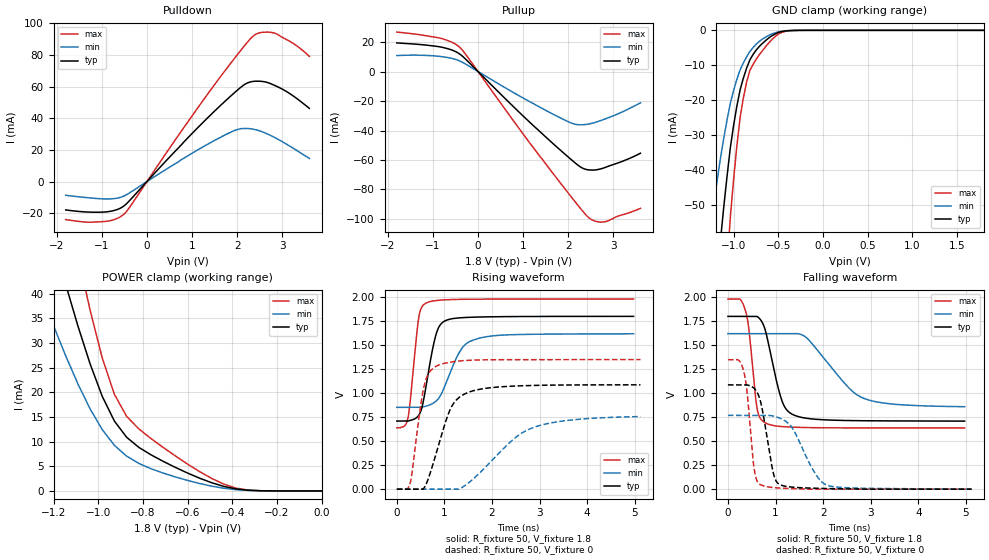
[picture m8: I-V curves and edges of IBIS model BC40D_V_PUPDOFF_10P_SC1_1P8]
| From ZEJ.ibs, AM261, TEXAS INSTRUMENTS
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[Model]   BC40D_V_PUPDOFF_10P_SC1_1P8
Model_type   I/O
Polarity   Non-Inverting
Enable   Active-Low
Vinl =  0.63
Vinh =  1.17
Cref =  15pF
Rref =  100.0000M
Vref =  0V
Vmeas =  0.9
C_comp   2.290246p   2.205796p   2.292736p
|[Input load] weak_pupdoff
|[Output drive] slow
|[supplytol] 10
|[temp] ind
[Model Spec]
Vinl   0.63   0.567   0.693
Vinh   1.17   1.053   1.287
[Temperature Range]   25   125   -40
[Voltage Range]   1.8   1.62   1.98
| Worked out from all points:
|   slope of the pulldown table from 0 to 0.27 V, typ, clamps not added: 32.2 ohm
|   slope of the pullup table from 0 to 0.27 V, typ, clamps not added: 32.6 ohm
|   GND clamp passes 1 mA (typ) near -0.53 V on its own axis
|   POWER clamp passes 1 mA (typ) near -0.44 V on its own axis
|   rising waveform, R_fixture 50, V_fixture 1.8: 20-80 % time 246ps typ, 417ps min, 160ps max; typ from 0.709 V to 1.8 V
|   rising waveform, R_fixture 50, V_fixture 0: 20-80 % time 429ps typ, 995ps min, 230ps max; typ from 0 V to 1.09 V
|   falling waveform, R_fixture 50, V_fixture 1.8: 20-80 % time 308ps typ, 788ps min, 165ps max; typ from 1.8 V to 0.709 V
|   falling waveform, R_fixture 50, V_fixture 0: 20-80 % time 226ps typ, 462ps min, 150ps max; typ from 1.09 V to 0 V
| Nom Voltages:
|   VDD=1.1001, VDDS=1.8, VDDS18=1.8, ESD_BIASFET=0, VSS=0, VSSS=0
| Min Voltages:
|   VDD=0.99, VDDS=1.62, VDDS18=1.62, ESD_BIASFET=0, VSS=0, VSSS=0
| Max Voltages:
|   VDD=1.21, VDDS=1.98, VDDS18=1.98, ESD_BIASFET=0, VSS=0, VSSS=0
[POWER_clamp]
|   voltage   I(typ)   I(min)   I(max)
-1.8V     158.8mA    112.5mA    219.7mA
-1.255V   59.93mA    40mA       84.85mA
-1.127V   39.08mA    25.51mA    55.74mA
-1.055V   28.36mA    18.34mA    40.4mA
-981.8mV  19.18mA    12.43mA    26.97mA
-927.3mV  14.16mA    9.242mA    19.58mA
-872.7mV  10.89mA    7.052mA    15.14mA
-818.2mV  8.843mA    5.581mA    12.58mA
-600mV    3.63mA     2.129mA    5.448mA
-436.4mV  903.9uA    539.1uA    1.358mA
-327.3mV  138.2uA    94.86uA    160.4uA
0V        19.3nA     120.3nA    352.8nA
[Pulldown]
|   voltage   I(typ)   I(min)   I(max)
-1.8V     -17.92mA   -8.674mA   -24.03mA
-927.3mV  -19.22mA   -10.99mA   -25.2mA
-654.5mV  -17.65mA   -10.46mA   -23.22mA
-490.9mV  -14.97mA   -8.904mA   -20.12mA
872.7mV   26.63mA    15.72mA    36.29mA
1.691V    49.7mA     28.87mA    68.59mA
2.127V    60.63mA    33.53mA    84.59mA
2.4V      63.43mA    32.84mA    92.9mA
2.564V    63.25mA    31.38mA    94.36mA
2.836V    60.69mA    27.76mA    93.76mA
3.273V    53.49mA    20.53mA    86.73mA
3.6V      46.26mA    14.64mA    79.12mA
[Pullup]
|   voltage   I(typ)   I(min)   I(max)
-1.8V     19.42mA    10.82mA    26.76mA
-818.2mV  16.58mA    10.15mA    22.47mA
-545.5mV  14.19mA    8.648mA    19.37mA
-381.8mV  11.34mA    6.842mA    15.75mA
1.036V    -31.26mA   -18.6mA    -43.9mA
1.909V    -55.59mA   -32.73mA   -78.89mA
2.182V    -62.72mA   -35.92mA   -89.47mA
2.345V    -65.94mA   -36.05mA   -95.62mA
2.455V    -66.75mA   -35.58mA   -99.18mA
2.618V    -66.67mA   -34.29mA   -101.7mA
2.836V    -64.85mA   -31.95mA   -101.8mA
3.6V      -55.4mA    -21.22mA   -92.82mA
[GND_clamp]
|   voltage   I(typ)   I(min)   I(max)
-1.8V     -270.2mA   -170.2mA   -430.1mA
-1.255V   -91.66mA   -55.91mA   -148.4mA
-1.145V   -59.91mA   -36.44mA   -97.09mA
-1.109V   -50.48mA   -30.83mA   -81.55mA
-1.073V   -41.73mA   -25.65mA   -67.05mA
-1.036V   -33.66mA   -20.92mA   -53.59mA
-927.3mV  -17.07mA   -11.35mA   -25.04mA
-854.5mV  -10.86mA   -7.616mA   -14.91mA
-781.8mV  -6.919mA   -4.945mA   -9.771mA
-636.4mV  -2.823mA   -1.868mA   -4.529mA
-381.8mV  -84.73uA   -78.7uA    -126.1uA
1.8V      19.3nA     3.129uA    310.3nA
[Ramp]
| variable   typ   min   max
dV/dt_f 0.66170168/0.31099039n 0.46782709/0.81087951n 0.81106408/0.16651847n
dV/dt_r 0.65944917/0.43266267n 0.47442459/1.0514017n 0.81583107/0.23074199n
R_load = 50
[Rising Waveform]
R_fixture = 50
V_fixture = 1.8
V_fixture_min = 1.62
V_fixture_max = 1.98
|   time   V(typ)   V(min)   V(max)
0s        709.3mV    852.1mV    638.8mV
228.2ps   709.3mV    852.1mV    728.2mV
277.2ps   715.1mV    852.1mV    895mV
458.2ps   767.3mV    852.1mV    1.778V
607.5ps   1.053V     863.6mV    1.936V
833.5ps   1.626V     920.9mV    1.965V
1.059ns   1.763V     1.136V     1.973V
1.377ns   1.786V     1.473V     1.978V
1.755ns   1.793V     1.575V     1.979V
4.974ns   1.8V       1.618V     1.98V
[Rising Waveform]
R_fixture = 50
V_fixture = 0
V_fixture_min = 0
V_fixture_max = 0
|   time   V(typ)   V(min)   V(max)
0s        0V         0V         0V
277.1ps   0V         0V         55.7mV
567ps     9.166mV    0V         1.061V
672.6ps   125mV      0V         1.208V
831.8ps   380.5mV    0V         1.282V
1.154ns   861.8mV    0V         1.325V
1.541ns   1.015V     79.05mV    1.343V
2.436ns   1.073V     513.7mV    1.349V
2.868ns   1.081V     641.9mV    1.349V
5.119ns   1.087V     756mV      1.349V
[Falling Waveform]
R_fixture = 50
V_fixture = 1.8
V_fixture_min = 1.62
V_fixture_max = 1.98
|   time   V(typ)   V(min)   V(max)
0s        1.8V       1.62V      1.981V
367.8ps   1.8V       1.62V      1.86V
439.5ps   1.8V       1.62V      1.67V
612.7ps   1.799V     1.62V      842.8mV
786.7ps   1.654V     1.62V      690.4mV
1.123ns   939.6mV    1.62V      652.7mV
1.375ns   774.7mV    1.62V      645.6mV
1.662ns   737.7mV    1.573V     641.7mV
2.828ns   713mV      952.2mV    638.2mV
4.974ns   709mV      859.5mV    637.9mV
[Falling Waveform]
R_fixture = 50
V_fixture = 0
V_fixture_min = 0
V_fixture_max = 0
|   time   V(typ)   V(min)   V(max)
0s        1.087V     768.8mV    1.349V
222.8ps   1.087V     768.8mV    1.344V
331.6ps   1.087V     768.8mV    1.228V
405.7ps   1.086V     768.8mV    997.5mV
555.4ps   1.048V     768.8mV    199.6mV
682.7ps   917.9mV    768.8mV    46.8mV
954.2ps   167.4mV    761.4mV    16.67mV
1.107ns   44.05mV    736.4mV    11.6mV
2.086ns   6.116mV    41.38mV    0V
5.119ns   0V         2.186mV    0V
